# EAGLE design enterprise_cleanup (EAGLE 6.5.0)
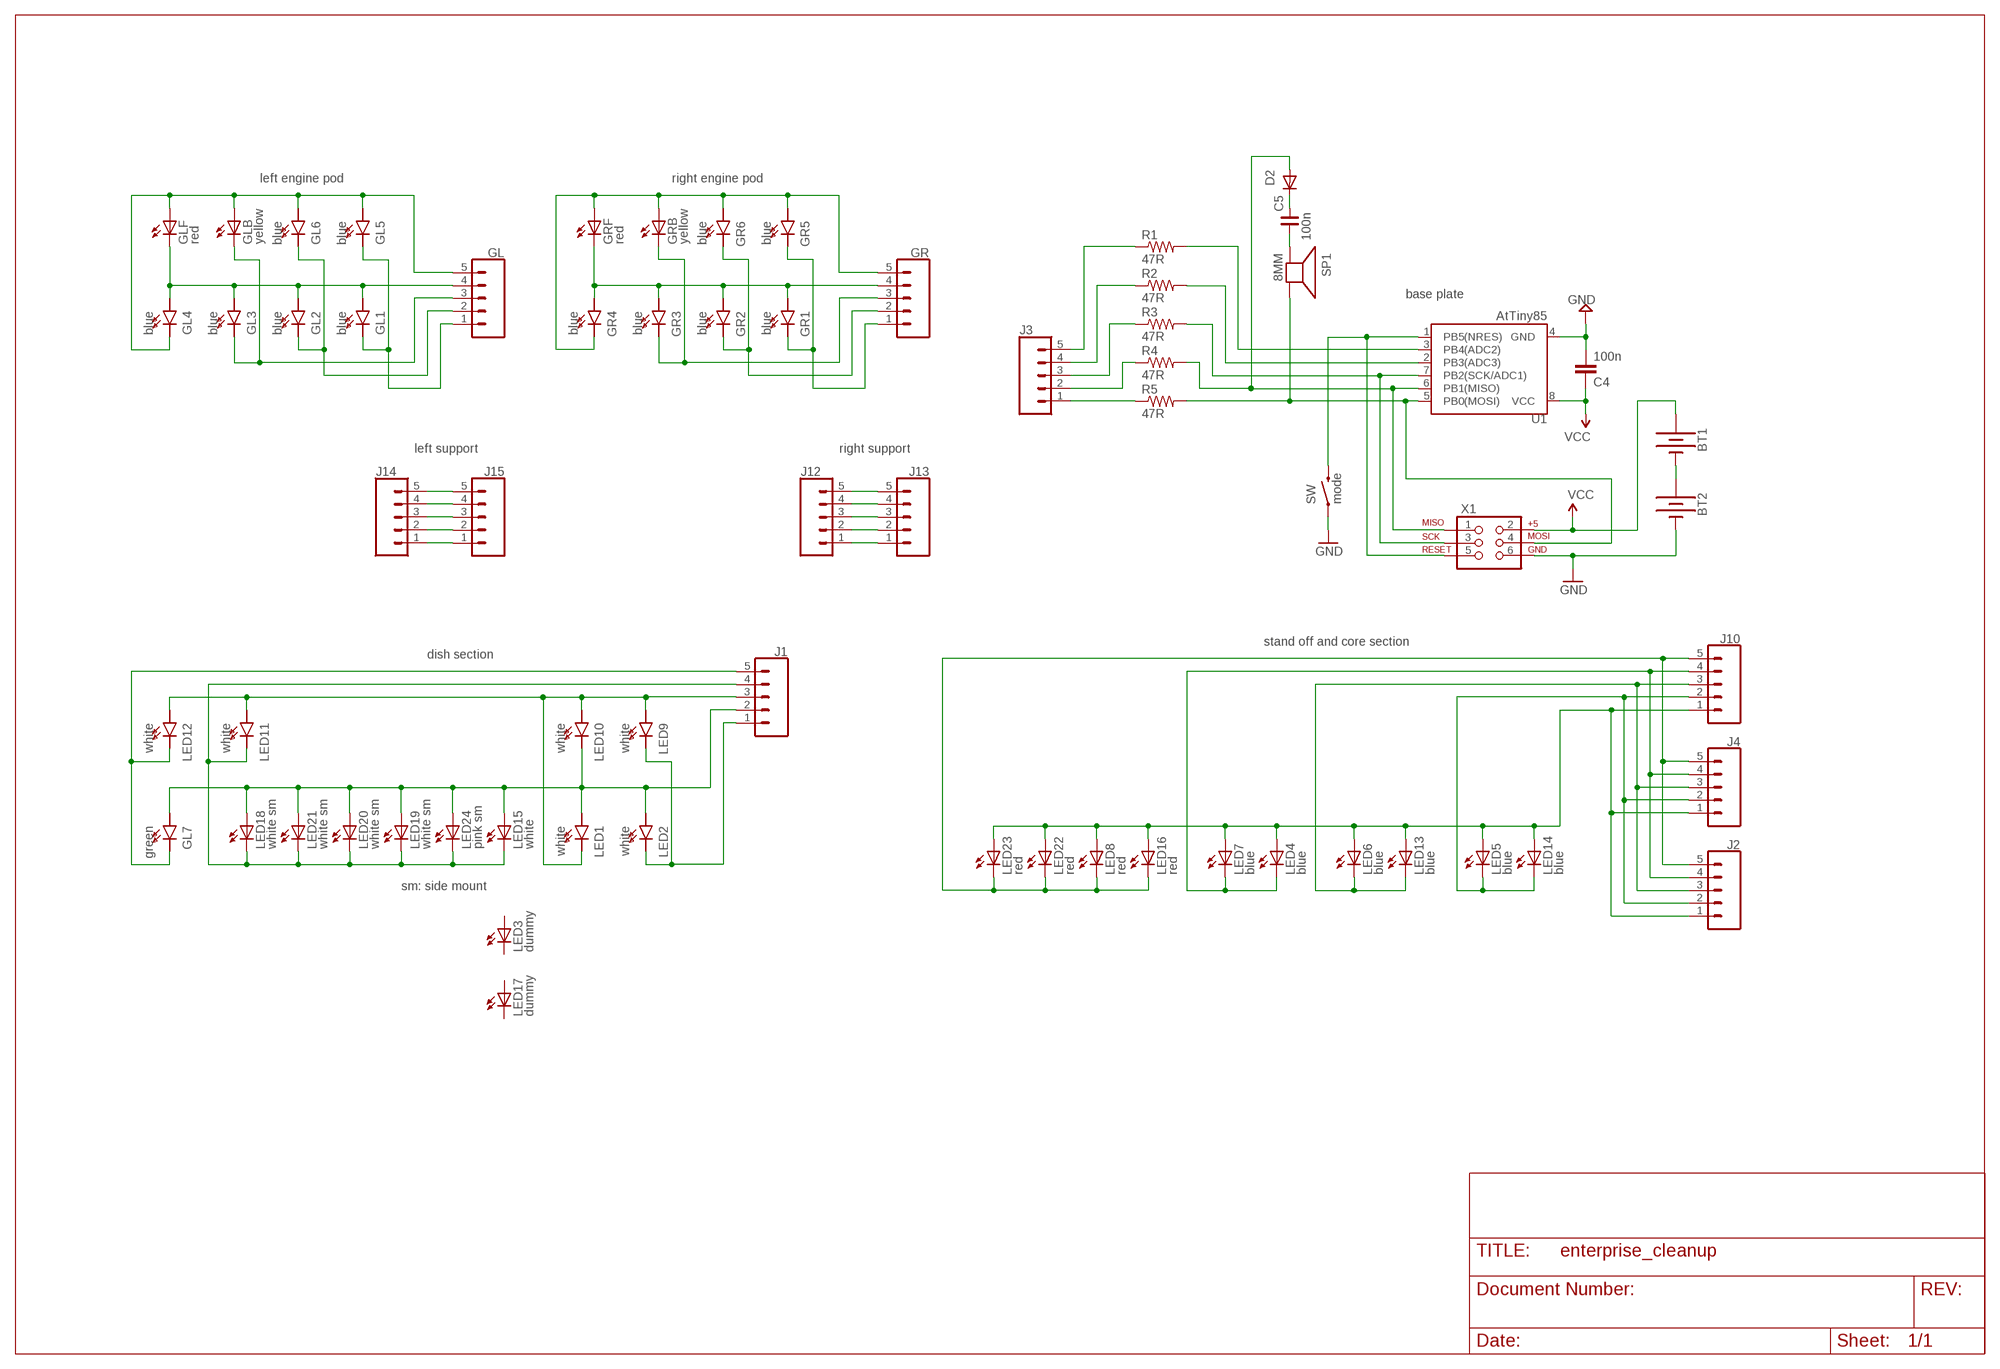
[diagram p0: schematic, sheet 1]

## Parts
BT1  BATTERY-AAA_KIT  [BATTERY-AAA-KIT]
BT2  BATTERY-AAA_KIT  [BATTERY-AAA-KIT]
C4  100n  CAP0603-CAP  [0603-CAP]
C5  100n  C_0603  [C0603]
D2  DIODESOD  [SOD-323]
GL  CONN_05NO_SILK  [1X05_NO_SILK]
GL1  blue  LED4014_SEGMENT3  [LED_4014_SEGMENT3]
GL2  blue  LED4014_SEGMENT3  [LED_4014_SEGMENT3]
GL3  blue  LED4014_SEGMENT3  [LED_4014_SEGMENT3]
GL4  blue  LED4014_SEGMENT3  [LED_4014_SEGMENT3]
GL5  blue  LED4014_SEGMENT3  [LED_4014_SEGMENT3]
GL6  blue  LED4014_SEGMENT3  [LED_4014_SEGMENT3]
GL7  green  LED4014_SEG_TRIANGLE  [LED_4014_SEGMENT2]
GLB  yellow  LEDCHIPLED_0805  [CHIPLED_0805]
GLF  red  LEDCHIPLED_0805  [CHIPLED_0805]
GR  CONN_05NO_SILK  [1X05_NO_SILK]
GR1  blue  LED4014_SEGMENT3  [LED_4014_SEGMENT3]
GR2  blue  LED4014_SEGMENT3  [LED_4014_SEGMENT3]
GR3  blue  LED4014_SEGMENT3  [LED_4014_SEGMENT3]
GR4  blue  LED4014_SEGMENT3  [LED_4014_SEGMENT3]
GR5  blue  LED4014_SEGMENT3  [LED_4014_SEGMENT3]
GR6  blue  LED4014_SEGMENT3  [LED_4014_SEGMENT3]
GRB  yellow  LEDCHIPLED_0805  [CHIPLED_0805]
GRF  red  LEDCHIPLED_0805  [CHIPLED_0805]
J1  CONN_05PTH_LONGPADS  [1X05_LONGPADS]
J2  CONN_05PTH_LONGPADS  [1X05_LONGPADS]
J3  CONN_05PTH_LONGPADS  [1X05_LONGPADS]
J4  CONN_05PTH_LONGPADS  [1X05_LONGPADS]
J10  CONN_05PTH_LONGPADS  [1X05_LONGPADS]
J12  CONN_05PTH_LONGPADS  [1X05_LONGPADS]
J13  CONN_05PTH_LONGPADS  [1X05_LONGPADS]
J14  CONN_05PTH_LONGPADS  [1X05_LONGPADS]
J15  CONN_05PTH_LONGPADS  [1X05_LONGPADS]
LED1  white  LED4014_SEGMENT3  [LED_4014_SEGMENT3]
LED2  white  LED4014_SEGMENT3  [LED_4014_SEGMENT3]
LED3  dummy  LED5MM  [LED5MM]
LED4  blue  LEDCHIPLED_0603  [CHIPLED_0603]
LED5  blue  LEDCHIPLED_0603  [CHIPLED_0603]
LED6  blue  LEDCHIPLED_0603  [CHIPLED_0603]
LED7  blue  LEDCHIPLED_0603  [CHIPLED_0603]
LED8  red  LEDCHIPLED_0805  [CHIPLED_0805]
LED9  white  LED4014_SEGMENT3  [LED_4014_SEGMENT3]
LED10  white  LED4014_SEGMENT3  [LED_4014_SEGMENT3]
LED11  white  LED4014_SEGMENT3  [LED_4014_SEGMENT3]
LED12  white  LED4014_SEGMENT3  [LED_4014_SEGMENT3]
LED13  blue  LEDCHIPLED_0603  [CHIPLED_0603]
LED14  blue  LEDCHIPLED_0603  [CHIPLED_0603]
LED15  white  LED5MM  [LED5MM]
LED16  red  LEDCHIPLED_0805  [CHIPLED_0805]
LED17  dummy  LED5MM  [LED5MM]
LED18  white sm  LEDCHIPLED_0805  [CHIPLED_0805]
LED19  white sm  LEDCHIPLED_0805  [CHIPLED_0805]
LED20  white sm  LEDCHIPLED_0805  [CHIPLED_0805]
LED21  white sm  LEDCHIPLED_0805  [CHIPLED_0805]
LED22  red  LEDCHIPLED_0805  [CHIPLED_0805]
LED23  red  LEDCHIPLED_0805  [CHIPLED_0805]
LED24  pink sm  LEDCHIPLED_0805  [CHIPLED_0805]
R1  47R  RESISTOR0603-RES  [0603-RES]
R2  47R  RESISTOR0603-RES  [0603-RES]
R3  47R  RESISTOR0603-RES  [0603-RES]
R4  47R  RESISTOR0603-RES  [0603-RES]
R5  47R  RESISTOR0603-RES  [0603-RES]
SP1  8MM  SPEAKER_BUZZER5MM  [BUZZER_SMT_5MM]
SW  mode  SWITCH-MOMENTARY-2SMD-3  [TACTILE_SWITCH_SMD-3]
U1  AtTiny85  ATTINY45TINY85-20-SMT  [SO08-EIAJ]
X1  AVR_SPI_PRG_6NS  [2X3-NS]

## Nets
E0: J2.1 J4.1 J10.1 LED4.A LED5.A LED6.A LED7.A LED8.A LED13.A LED14.A LED16.A LED22.A LED23.A
E1: J2.2 J4.2 J10.2 LED5.C LED14.C
E2: J2.3 J4.3 J10.3 LED6.C LED13.C
E3: J2.4 J4.4 J10.4 LED4.C LED7.C
E4: J2.5 J4.5 J10.5 LED8.C LED16.C LED22.C LED23.C
G0: GL1.K(C) GL5.K(C) GL.1
G1: GL2.K(C) GL6.K(C) GL.2
G2: GL3.K(C) GL.3 GLB.C
G3: GL1.A GL2.A GL3.A GL4.A GL.4 GLF.C
G4: GL4.K(C) GL5.A GL6.A GL.5 GLB.A GLF.A
GND: BT2.GND@1(-) C4.2 SW.1 U1.4(GND) X1.6
LX1: J3.1 R5.1
LX2: J3.2 R4.1
LX3: J3.3 R3.1
LX4: J3.4 R2.1
LX5: J3.5 R1.1
N$2: BT1.GND@1(-) BT2.PWR@1(+)
N$4: J12.1 J13.1
N$11: J12.2 J13.2
N$12: J12.3 J13.3
N$13: J12.4 J13.4
N$14: J12.5 J13.5
N$15: J14.1 J15.1
N$16: J14.2 J15.2
N$17: J14.3 J15.3
N$18: J14.4 J15.4
N$19: J14.5 J15.5
N$20: C5.2 D2.1(C)
N$21: C5.1 SP1.+
N$27: GR4.K(C) GR5.A GR6.A GR.5 GRB.A GRF.A
N$28: GR1.A GR2.A GR3.A GR4.A GR.4 GRF.C
N$29: GR3.K(C) GR.3 GRB.C
N$30: GR2.K(C) GR6.K(C) GR.2
N$31: GR1.K(C) GR5.K(C) GR.1
PB0: R5.2 SP1.- U1.5(PB0(MOSI)) X1.4
PB1: D2.2(A) R4.2 U1.6(PB1(MISO)) X1.1
PB2: R3.2 U1.7(PB2(SCK/ADC1)) X1.3
PB3: R2.2 U1.2(PB3(ADC3))
PB4: R1.2 U1.3(PB4(ADC2))
RESET: SW.4 U1.1(PB5(NRES)) X1.5
T0: J1.1 LED2.K(C) LED9.K(C)
T1: GL7.A J1.2 LED1.A LED2.A LED10.K(C) LED15.A LED18.A LED19.A LED20.A LED21.A LED24.A
T2: J1.3 LED1.K(C) LED9.A LED10.A LED11.A LED12.A
T3: J1.4 LED11.K(C) LED15.K(C) LED18.C LED19.C LED20.C LED21.C LED24.C
T4: GL7.K(C) J1.5 LED12.K(C)
VCC [pwr]: BT1.PWR@1(+) C4.1 U1.8(VCC) X1.2
Unconnected: LED3.A LED3.K(C) LED17.A LED17.K(C)

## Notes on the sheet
- left engine pod | right engine pod
- base plate
- left support | right support
- stand off and core section
- dish section
- sm: side mount

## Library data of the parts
BT1 BT2 = SparkFun-Batteries:BATTERY: Battery - Single Cell; PROD_ID: BATT-08571; SF_SKU: PRT-12718
C4 = SparkFun:CAP: Capacitor
C5 = rc-master-smd:C_: NON-POLARIZED CAP
D2 = SparkFun:DIODE: Diode
GL GR J1-J4 J10 J12-J15 = SparkFun-Connectors:CONN_05: Multi connection point. Often used as Generic Header-pin footprint for 0.1 inch spaced/style header connections On any of the 0.1 inch spaced packages, you can populate with these: Break Away Headers - Straight (PRT-00116) Break Away Male Headers - Right Angle (PRT-00553) Female Headers (PRT-00115)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
GL1-GL7 GR1-GR6 LED1 LED2 LED9-LED12 = yg_custom.5.5:LED
GLB GLF GRB GRF LED3-LED8 LED13-LED24 = led:LED: LED
R1-R5 = SparkFun:RESISTOR: Resistor
SP1 = microbuilder:SPEAKER: SPEAKER
SW = SparkFun-Electromechanical:SWITCH-MOMENTARY-2: Various NO switches- pushbuttons, reed, etc
U1 = SparkFun-DigitalIC:ATTINY45: Atmel 8-pin 2/4/8kB flash uC; PROD_ID: IC-09092; VALUE: Tiny85-20-SMT
X1 = SparkFun:AVR_SPI_PRG_6: AVR ISP 6 Pin This is the reduced ISP connector for AVR programming. Common on Arduino. This footprint will take up less PCB space and can be used with a 10-pin to 6-pin adapter such as SKU: BOB-08508

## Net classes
0 default: width 0.254 mm, drill 0.356 mm, clearance 0.381 mm
1 GNDa: width 0.254 mm, drill 0.356 mm, clearance 0.381 mm
2 pwr: width 0.254 mm, drill 0.356 mm, clearance 0.381 mm

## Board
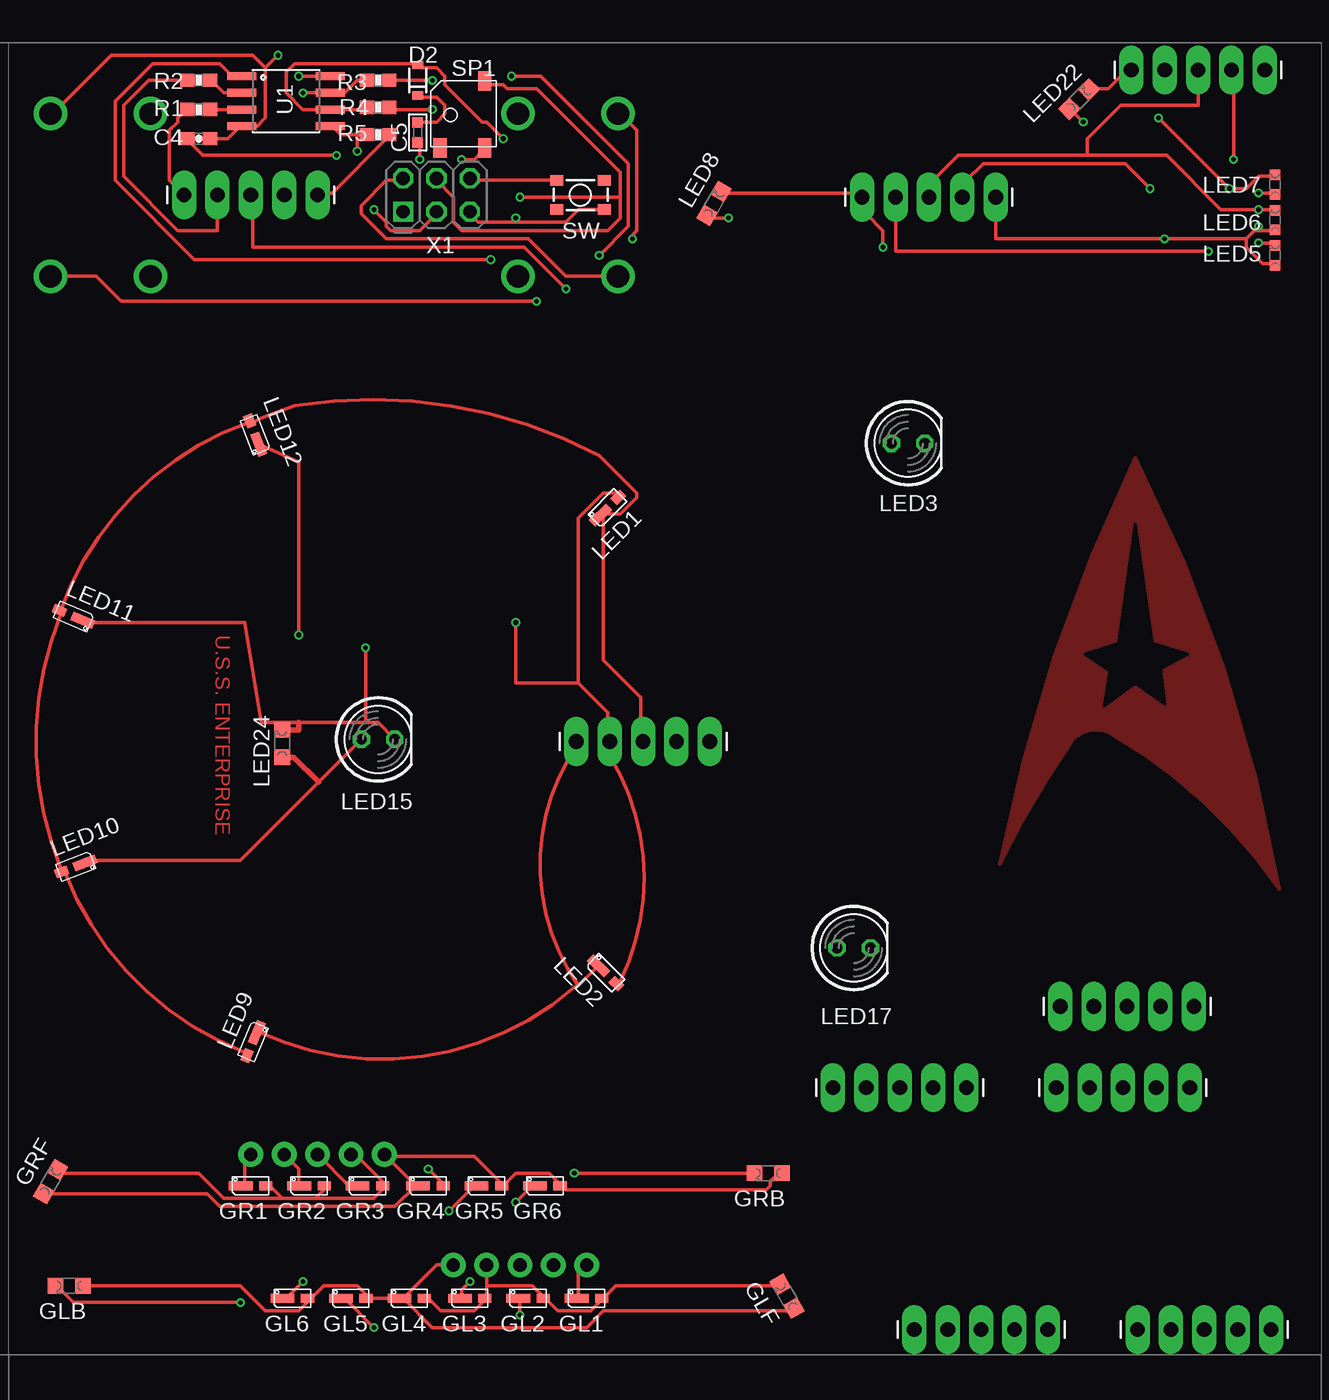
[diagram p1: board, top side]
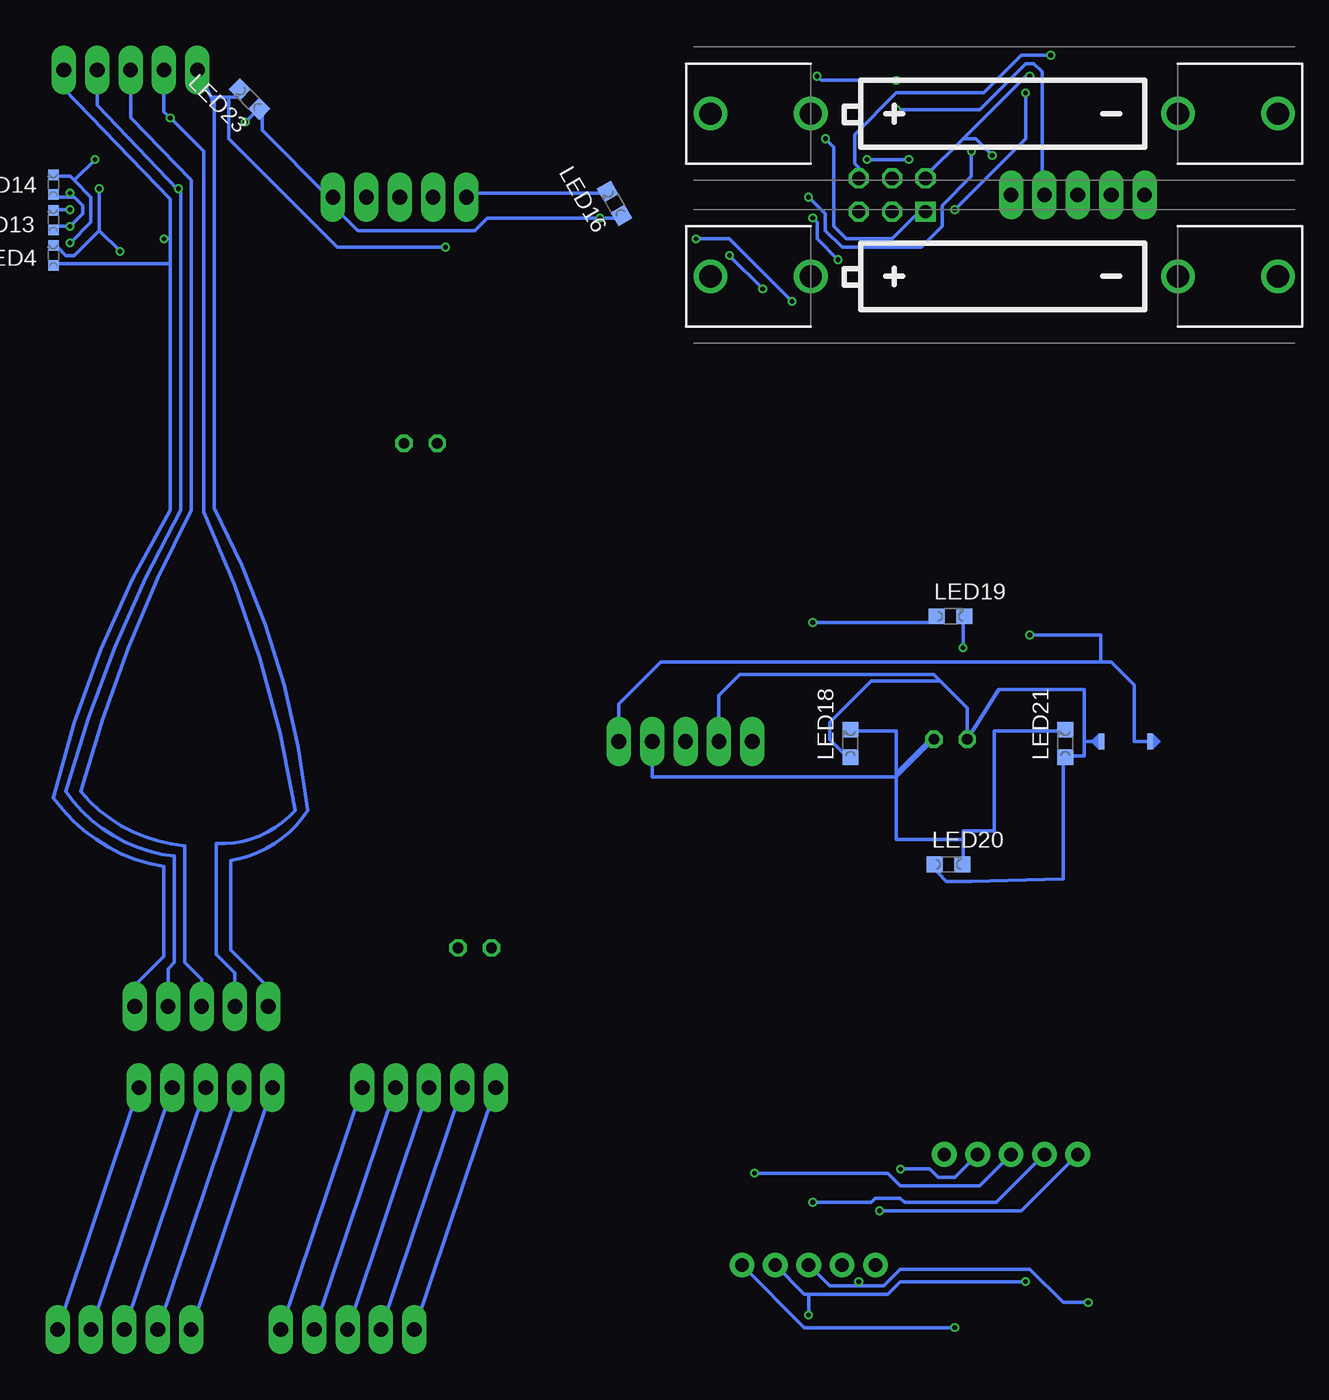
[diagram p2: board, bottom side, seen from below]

No outline drawn. Coordinates in mm, seen from the top.
Copper layers (1*16): Top 0.035mm / dielectric 1.5mm / Bottom 0.035mm
Design rules "ITEADstudio_DRC *": minimum track width 6mil, minimum drill 12mil, track to track 6mil, track to pad 6mil, pad to pad 6mil, via to via 6mil, smd to smd 0mil, copper to edge 20mil, drill to drill 8mil, minimum pad ring 10mil, minimum via ring 6mil, stop-mask expansion 2mil, vias tented up to drill 100mil, thermal gap 10mil
tRestrict: area 187.5,72.4 to 195.3,86.2

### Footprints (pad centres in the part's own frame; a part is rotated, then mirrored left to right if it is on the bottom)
BATTERY-AAA-KIT = drill 1.702: GND@1 21.59,0; GND@2 13.97,0; PWR@1 -21.59,0; PWR@2 -13.97,0
0603-CAP = smd 1.1 x 1: 1 -0.85,0; 2 0.85,0
C0603 = smd 0.8 x 0.8: 1 -0.762,0; 2 0.762,0
SOD-323 = smd 0.63 x 0.83: 1 -1.15,0; 2 1.15,0
1X05_NO_SILK = drill 1.016 pad 1.88: 1 0,0; 2 2.54,0; 3 5.08,0; 4 7.62,0; 5 10.16,0
LED_4014_SEGMENT3 = smd 1 x 0.7: A -1.143,0 | smd 1.8 x 0.7: K 0.762,0
LED_4014_SEGMENT2 = smd 0.4 x 1.2: A -1.85,0; K 1.85,0
CHIPLED_0805 = smd 1.2 x 1.2: A 0,-1.05; C 0,1.05
1X05_LONGPADS = drill 1.118 pad 1.88 long: 1 0,0; 2 2.54,0; 3 5.08,0; 4 7.62,0; 5 10.16,0
LED5MM = drill 0.813 octagon: A -1.27,0; K 1.27,0
CHIPLED_0603 = smd 0.8 x 0.8: A 0,-0.75; C 0,0.75
0603-RES = smd 1.1 x 1: 1 -0.85,0; 2 0.85,0
BUZZER_SMT_5MM = smd 1.5 x 1: + -2.6,-1.6; - 2.5,-1.6; MT -2.6,1.8
TACTILE_SWITCH_SMD-3 = smd 1 x 0.8: 1 -1.8,1.1; 2 1.8,1.1; 3 -1.8,-1.1; 4 1.8,-1.1
SO08-EIAJ = smd 0.61 x 2.21: 1 -1.905,-3.378; 2 -0.635,-3.378; 3 0.635,-3.378; 4 1.905,-3.378; 5 1.905,3.353; 6 0.635,3.353; 7 -0.635,3.353; 8 -1.905,3.353
2X3-NS = drill 1.016 square: 1 -2.54,-1.27 | drill 1.016 octagon: 2 -2.54,1.27; 3 0,-1.27; 4 0,1.27; 5 2.54,-1.27; 6 2.54,1.27

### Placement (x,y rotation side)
BT1  130.33,105.09 0 bottom
BT2  130.33,117.47 0 bottom
C4  120.02,115.57 0 top
C5  136.68,116.05 90 top
D2  136.68,120.02 90 top
GL  149.54,29.84 0 bottom
GL1  149.54,27.3 180 top
GL2  145.1,27.3 180 top
GL3  140.65,27.3 180 top
GL4  136.05,27.3 180 top
GL5  131.6,27.3 180 top
GL6  127.16,27.3 180 top
GL7  120.33,69.69 0 bottom
GLB  110.17,28.26 90 top
GLF  164.78,27.46 30 top
GR  123.98,38.26 0 top
GR1  123.98,35.88 180 top
GR2  128.43,35.88 180 top
GR3  132.87,35.88 180 top
GR4  137.48,35.88 180 top
GR5  141.92,35.88 180 top
GR6  146.37,35.88 180 top
GRB  163.35,36.83 90 top
GRF  108.74,36.2 330 top
J1  148.75,69.69 0 top
J2  195.74,49.53 180 top
J3  129.06,111.28 180 top
J4  180.66,111.12 180 top
J10  201.14,120.81 180 top
J12  201.61,24.92 180 top
J13  195.42,43.34 180 top
J14  184.63,24.92 180 top
J15  178.44,43.34 180 top
LED1  151.13,87.47 225 top
LED2  150.97,52.07 135 top
LED3  173.99,92.39 0 top
LED4  201.93,106.68 0 bottom
LED5  201.93,106.68 0 top
LED6  201.93,109.38 0 top
LED7  201.93,112.08 0 top
LED8  159.23,110.65 330 top
LED9  124.14,46.83 67 top
LED10  110.65,60.17 21 top
LED11  110.49,79.22 337 top
LED12  124.3,93.03 291 top
LED13  201.93,109.38 0 bottom
LED14  201.93,112.08 0 bottom
LED15  133.67,69.85 0 top
LED16  159.23,110.65 30 bottom
LED17  169.86,53.98 0 top
LED18  141.29,69.53 0 bottom
LED19  133.67,79.22 270 bottom
LED20  133.83,60.33 270 bottom
LED21  124.94,69.53 0 bottom
LED22  187.01,118.59 315 top
LED23  187.01,118.59 45 bottom
LED24  126.36,69.53 0 top
R1  120.02,117.79 0 top
R2  120.02,120.02 0 top
R3  133.67,120.02 180 top
R4  133.67,117.95 180 top
R5  133.67,115.89 180 top
SP1  140.18,117.47 90 top
SW  149.07,111.28 0 top
U1  126.68,118.43 270 top
U$1  [A4L-LOC]  34.13,-28.26 0 top
X1  138.11,111.28 0 top

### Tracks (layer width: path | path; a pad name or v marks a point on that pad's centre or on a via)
E0  (via drill 0.36)
  Top 0.254: v200.66,111.44 201.93,111.44 LED14.A | 199.71,107.95 199.71,107.31 200.98,106.05 201.93,106.05 LED4.A | 199.71,107.95 200.34,108.58 200.66,108.58 | 200.66,108.58 201.93,108.58 LED13.A | v160.34,109.54 158.43,109.54 LED16.A | 199.71,107.95 v193.52,107.95 180.66,107.95 J4.1 | 200.66,108.58 v200.66,108.9 | v187.32,116.84 186.69,117.47 LED23.A
  Bottom 0.254: J2.1 195.74,51.12 193.52,53.34 193.52,60.17 arc45 201.93,65.41 arc17 193.04,87.31 193.04,106.05 | 193.04,106.05 193.04,107.95 | 193.04,107.95 193.04,110.97 201.14,119.38 J10.1 | 193.04,106.05 201.93,106.05 LED4.A | 200.66,111.12 201.93,111.12 LED14.A | 200.66,111.12 200.34,111.12 199.71,110.49 199.71,109.86 v200.66,108.9 201.93,108.9 LED13.A | 200.66,111.12 v200.66,111.44 | v160.34,109.54 158.43,109.54 LED16.A 158.75,109.54 168.91,109.54 169.86,108.58 178.75,108.58 180.66,110.49 J4.1 180.97,111.12 186.06,116.2 186.06,117.47 LED23.A 186.69,117.47 v187.32,116.84 | v193.52,107.95 193.04,107.95
E1  (via drill 0.36)
  Top 0.254: v200.66,107.63 201.93,107.63 LED5.C | v198.75,113.98 198.75,120.65 J10.2 | v192.41,111.76 190.5,113.67 179.71,113.67 178.44,112.39 178.44,111.12 J4.2
  Bottom 0.254: J2.2 193.2,52.39 192.72,52.86 192.72,60.96 arc49 200.98,65.88 arc14 192.25,87.31 192.25,111.44 192.48,111.69 | 192.48,111.69 198.6,118.11 J10.2 | v200.66,107.63 199.07,109.22 199.07,111.12 200.34,112.39 | 200.34,112.39 200.66,112.71 201.93,112.71 LED14.C | v198.75,113.98 200.34,112.39 | v192.41,111.76 192.48,111.69
E2  (via drill 0.36)
  Top 0.254: LED13.C 201.93,110.17 v200.66,110.17 197.8,110.17 193.68,114.3 187.64,114.3 | 187.64,114.3 187.64,115.57 190.18,118.11 196.06,118.11 J10.3 | 187.64,114.3 177.8,114.3 175.9,112.39 175.9,111.12 J4.3
  Bottom 0.254: J2.3 190.66,51.59 191.93,52.86 191.93,61.75 arc45 199.87,65.88 arc12 191.45,87.31 191.45,112.39 196.06,117.16 J10.3 | v200.66,110.17 201.93,110.17 LED13.C
E3  (via drill 0.36)
  Top 0.254: LED7.C 201.93,112.71 200.66,112.71 199.71,111.76 v198.44,111.76 v193.04,117.16 | J4.4 173.04,107 v196.85,107
  Bottom 0.254: J2.4 188.12,52.07 189.55,53.5 189.55,61.91 arc-51 183.51,64.45 arc-16 190.5,87.15 190.5,114.62 v193.04,117.16 193.52,117.63 J10.4 | 198.44,108.58 200.34,106.68 200.98,106.68 201.61,107.31 201.93,107.31 LED4.C | v198.44,111.76 198.44,108.58 | 198.44,108.58 v196.85,107
E4  (via drill 0.36)
  Top 0.254: LED16.C 160.02,111.44 170.18,111.44 J4.5 170.81,111.12 170.81,109.86 172.09,108.58 v172.09,107.31 | LED23.C 187.96,119.38 189.23,119.38 190.5,120.65 J10.5
  Bottom 0.254: J2.5 185.58,50.96 188.44,53.82 188.44,60.64 arc-48 182.56,64.45 arc-22 189.71,87.47 189.71,118.27 189.8,118.46 | 189.8,118.46 189.93,118.71 | 189.93,118.71 J10.5 | LED16.C 160.02,111.44 170.18,111.44 J4.5 | 189.87,118.43 189.8,118.46 | 188.59,118.75 189.87,118.75 189.93,118.71 | 188.59,118.75 187.96,118.75 LED23.C | 188.59,118.75 188.59,115.57 180.34,107.31 v172.09,107.31
G0  (via drill 0.36)
  Top 0.254: v133.35,25.08 131.13,27.3 GL5.K | GL.1 148.91,29.21 148.91,27.3 GL1.K
  Bottom 0.254: v133.35,25.08 144.78,25.08 GL.1
G1  (via drill 0.36)
  Top 0.254: v127.95,28.57 126.68,27.3 GL6.K | v144.46,26.04 144.46,27.3 GL2.K
  Bottom 0.254: v127.95,28.57 137.48,28.57 138.43,27.62 144.46,27.62 | 144.46,27.62 144.78,27.62 GL.2 | 144.46,27.62 v144.46,26.04
G2  (via drill 0.36)
  Top 0.254: v123.19,26.99 110.49,26.99 109.22,28.26 GLB.C | v140.65,28.57 140.02,27.94 140.02,27.3 GL3.K
  Bottom 0.254: v123.19,26.99 125.09,26.99 127.64,29.53 137.48,29.53 138.75,28.26 140.65,28.26 | 140.65,28.26 142.88,28.26 GL.3 | 140.65,28.26 v140.65,28.57
G3
  Top 0.254: 141.92,27.3 140.97,26.35 138.43,26.35 137.48,27.3 GL4.A | GL.4 141.92,28.26 | 141.92,28.26 141.92,27.3 | 141.92,27.3 GL3.A | 146.37,27.3 147.32,26.35 149.86,26.35 150.81,27.3 | 150.81,27.3 151.76,28.26 164.15,28.26 GLF.C | 150.81,27.3 GL1.A | 141.92,28.26 145.41,28.26 146.37,27.3 | 146.37,27.3 GL2.A
G4
  Top 0.254: 128.59,27.3 129.54,28.26 132.08,28.26 133.03,27.3 | GLB.A 123.19,28.26 125.09,26.35 127.64,26.35 128.59,27.3 | 128.59,27.3 GL6.A | 135.57,27.3 137.79,25.08 149.54,25.08 150.81,26.35 165.1,26.35 GLF.A | GL.5 138.11,29.84 135.57,27.3 | 135.57,27.3 GL4.K 133.03,27.3 | 133.03,27.3 GL5.A
GND  (via drill 0.36)
  Top 0.254: SW.1 147,112.39 140.65,112.39 X1.6 | C4.2 122.24,115.57 123.19,116.52 U1.4 124.46,116.52 125.09,117.16 125.09,120.97 | 125.09,120.97 124.14,121.92 113.35,121.92 108.9,117.47 BT2.GND@1 | 125.09,120.97 v126.05,121.92
  Bottom 0.254: X1.6 140.65,113.35 140.97,113.67 140.97,115.89 137.79,119.06 131.13,119.06 128.27,121.92 v126.05,121.92
LX1
  Top 0.254: R5.1 134.3,115.89 134.3,115.57 130.18,111.44 129.22,111.44 J3.1
LX2  (via drill 0.36)
  Top 0.254: v137.79,117.79 134.62,117.79 R4.1
  Bottom 0.254: v137.79,117.79 131.44,117.79 127.95,121.28 127.32,121.28 126.68,120.65 126.68,111.44 J3.2
LX3  (via drill 0.36)
  Top 0.254: v137.79,120.02 R3.1 | v143.83,120.33 146.05,120.33 152.72,113.67 152.72,108.9 v150.5,106.68 | v147.96,104.14 144.78,107.31 124.14,107.31 124.14,111.12 J3.3
  Bottom 0.254: v137.79,120.02 143.51,120.02 v143.83,120.33 | v147.96,104.14 v150.5,106.68
LX4
  Top 0.254: R2.1 116.2,120.02 114.3,118.11 114.3,112.71 118.43,108.58 121.44,108.58 J3.4
LX5
  Top 0.254: J3.5 117.79,112.39 117.79,116.2 118.43,116.84 118.43,117.16 119.06,117.79 R1.1
N$2  (via drill 0.36)
  Top 0.254: BT1.GND@1 112.24,105.09 114.14,103.19 v145.73,103.19 | v153.03,107.95 153.03,108.27 153.35,108.58 153.35,116.2 152.08,117.47 BT2.PWR@1
  Bottom 0.254: v145.73,103.19 150.5,107.95 v153.03,107.95
N$4
  Bottom 0.254: J12.1 J13.1
N$9
  pour Top: 180.97,60.33 arc-15 191.29,91.28 arc-17 202.25,58.42 arc25 189.39,70.33 arc70 186.53,69.85 arc9
N$11
  Bottom 0.254: J12.2 J13.2
N$12
  Bottom 0.254: J12.3 J13.3
N$13
  Bottom 0.254: J12.4 J13.4
N$14
  Bottom 0.254: J12.5 J13.5
N$15
  Bottom 0.254: J14.1 J15.1
N$16
  Bottom 0.254: J14.2 J15.2
N$17
  Bottom 0.254: J14.3 J15.3
N$18
  Bottom 0.254: J14.4 J15.4
N$19
  Bottom 0.254: J14.5 J15.5
N$20
  Top 0.254: C5.2 136.84,116.84 138.11,116.84 138.75,117.47 138.75,118.11 138.11,118.75 136.84,118.75 D2.1
N$21  (via drill 0.36)
  Top 0.254: v136.84,113.98 136.84,115.25 C5.1 | v140.02,113.98 140.97,113.98 141.6,114.62 SP1.+
  Bottom 0.254: v140.02,113.98 v136.84,113.98
N$27
  Top 0.254: 147.64,35.88 146.69,36.83 144.15,36.83 143.19,35.88 GR5.A 142.88,35.88 142.88,36.2 140.97,38.1 134.3,38.1 | 147.64,35.88 147.96,35.56 163.19,35.56 163.51,35.88 163.51,36.2 164.15,36.83 GRB.A | 147.64,35.88 GR6.A | 136.53,35.88 134.94,34.29 121.6,34.29 120.65,35.24 108.27,35.24 GRF.A | 136.53,35.88 134.3,38.1 | 136.53,35.88 GR4.K | 134.3,38.1 GR.5
N$28  (via drill 0.36)
  Top 0.254: 133.99,35.88 133.99,36.2 131.76,38.42 GR.4 | v137.48,37.15 138.43,36.2 138.43,35.88 GR4.A | 126.36,34.92 125.41,35.88 GR1.A | 128.91,34.92 126.36,34.92 | 128.91,34.92 129.86,35.88 GR2.A | 126.36,34.92 121.92,34.92 120.02,36.83 109.54,36.83 GRF.C | 133.99,35.88 133.99,35.56 133.35,34.92 128.91,34.92 | 133.99,35.88 GR3.A
  Bottom 0.254: v137.48,37.15 135.25,37.15 134.62,36.51 133.35,36.51 GR.4
N$29  (via drill 0.36)
  Top 0.254: v148.59,36.83 GRB.C | GR3.K 131.44,35.88 GR.3
  Bottom 0.254: v148.59,36.83 138.43,36.83 137.48,35.88 131.44,35.88 GR.3
N$30  (via drill 0.36)
  Top 0.254: GR.2 127.64,37.15 127.64,35.88 GR2.K | v144.15,34.61 145.41,35.88 GR6.K
  Bottom 0.254: v144.15,34.61 139.7,34.61 139.38,34.92 137.48,34.92 137.16,34.61 130.18,34.61 GR.2
N$31  (via drill 0.36)
  Top 0.254: GR.1 123.51,37.78 123.51,35.88 GR1.K | v139.06,33.97 140.97,35.88 GR5.K
  Bottom 0.254: v139.06,33.97 128.27,33.97 GR.1
PB0  (via drill 0.36)
  Top 0.254: 132.08,115.89 130.81,115.89 130.18,116.52 U1.5 | 132.08,115.89 R5.2 | 152.08,111.12 152.08,109.54 151.13,108.58 140.02,108.58 139.38,109.22 139.38,111.12 138.11,112.39 X1.4 | 152.08,111.12 152.08,113.03 145.73,119.38 143.51,119.38 143.19,119.7 141.92,119.7 SP1.- | v132.08,114.62 132.08,115.89 | 152.08,111.12 v144.46,111.12
  Bottom 0.254: v132.08,114.62 132.08,112.71 134.3,110.49 134.3,108.9 135.89,107.31 141.92,107.31 143.19,108.58 143.19,109.86 v144.46,111.12
PB1  (via drill 0.36)
  Top 0.254: R4.2 132.72,117.79 U1.6 127.95,117.79 126.68,119.06 126.68,120.65 127.32,121.28 136.53,121.28 D2.2 136.84,120.97 138.11,120.97 138.75,120.33 138.75,119.7 141.6,116.84 141.92,116.84 v143.19,115.57
  Bottom 0.254: v143.19,115.57 142.56,114.94 142.56,108.9 141.6,107.95 138.11,107.95 136.21,109.86 135.57,109.86 X1.1
PB2  (via drill 0.36)
  Top 0.254: R3.2 132.08,120.02 131.13,119.06 U1.7 v127.95,119.06 | v133.35,110.17 134.3,109.22 134.3,108.9 134.62,108.58 136.84,108.58 138.11,109.86 X1.3
  Bottom 0.254: v127.95,119.06 127.95,115.57 v133.35,110.17
PB3
  Top 0.254: U1.2 121.92,119.06 120.97,120.02 R2.2
PB4
  Top 0.254: U1.3 R1.2
RESET  (via drill 0.36)
  Top 0.254: 144.15,109.22 141.29,109.22 140.65,109.86 X1.5 | 144.15,109.22 147.96,109.22 148.91,110.17 150.81,110.17 SW.4 | U1.1 122.56,120.33 121.6,121.28 116.52,121.28 113.67,118.43 113.67,112.39 119.7,106.36 v142.24,106.36 | 144.15,109.22 v144.15,109.54
  Bottom 0.254: v142.24,106.36 143.83,107.95 143.83,109.22 v144.15,109.54
T0
  Top 0.254: 148.91,51.12 150.18,52.39 LED2.K | 148.91,51.12 148.59,50.96 arc-66 124.46,47.62 LED9.K | 148.91,51.12 arc-70 148.91,69.53 J1.1
T1  (via drill 0.36)
  Top 0.254: LED2.A 152.08,51.44 arc58 151.29,68.58 J1.2 151.13,69.85 151.13,71.91 148.91,74.14 | 148.91,74.14 148.91,86.68 150.81,88.58 151.76,88.58 LED1.A | LED15.A 129.14,66.6 123.19,60.64 111.44,60.64 LED10.K | 148.91,74.14 144.15,74.14 v144.15,78.74
  Top 0.406: LED24.A 127.26,68.48 129.14,66.6
  Bottom 0.254: GL7.A 123.51,69.69 | 134.54,74.37 132.4,72.23 LED15.A 130.02,73.66 123.51,73.66 123.51,69.69 | 134.54,74.37 134.94,74.77 149.7,74.77 151.29,73.18 J1.2 | 123.51,69.69 123.51,68.58 124.46,68.58 LED21.A 125.09,67.94 125.09,59.21 132.08,59.05 133.99,59.05 134.62,59.69 134.62,60.33 LED20.A | v144.15,78.74 135.25,78.74 LED19.A | LED18.A 141.6,68.58 142.88,69.85 142.88,71.12 139.7,74.3 134.62,74.3 134.54,74.37
T2
  Top 0.254: J1.3 153.67,69.85 153.67,73.03 150.81,75.88 150.81,86.68 LED1.K 150.81,87 152.08,87 153.35,88.27 153.35,88.58 150.5,91.44 arc37 127.32,95.25 124.78,94.3 124.14,93.98 LED12.A 123.83,93.98 arc51 109.54,79.69 LED11.A 109.54,79.38 arc45 109.54,60.01 LED10.A 109.86,59.69 arc47 123.51,46.04 LED9.A
T3  (via drill 0.36)
  Top 0.254: 132.72,71.12 133.67,71.12 LED15.K | 132.72,71.12 127.64,71.12 124.78,71.12 123.51,78.74 111.44,78.74 LED11.K | 132.72,71.12 v132.72,76.83
  Top 0.406: LED24.C 127.64,70.58 127.64,71.12
  Bottom 0.254: J1.4 156.37,66.99 137.79,66.99 LED15.K 135.25,69.85 137.79,67.31 | v132.72,76.83 132.72,78.74 LED19.C | 132.72,62.23 132.72,60.33 LED20.C | 132.72,62.23 132.72,62.87 130.33,62.87 130.33,70.48 125.09,70.48 LED21.C | 132.72,62.23 137.79,62.23 137.79,67.31 | 137.79,67.31 137.79,70.48 140.97,70.48 LED18.C
T4  (via drill 0.36)
  Top 0.254: v127.64,77.79 127.64,90.96 LED12.K
  Bottom 0.254: GL7.K 119.7,69.69 119.7,73.98 121.44,75.72 122.24,75.72 | 122.24,75.72 155.73,75.72 158.91,72.55 J1.5 | v127.64,77.79 122.24,77.79 122.24,75.72
VCC  (via drill 0.36)
  Top 0.254: v130.49,114.3 120.33,114.3 119.38,115.25 119.38,115.57 C4.1 | v127.64,120.33 U1.8 | BT1.PWR@1 147.96,105.09 145.1,107.95 134.3,107.95 132.4,109.86 132.4,110.49 134.3,112.39 135.57,112.39 X1.2
  Bottom 0.254: v130.49,114.3 131.76,115.57 132.72,115.57 | 132.72,115.57 135.57,112.71 X1.2 | v127.64,120.33 127.95,120.33 132.72,115.57

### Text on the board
Top: U.S.S. ENTERPRISE
tStop: U.S.S. ENTERPRISE
t_draw: boldly go ... | ENGAGE | U.S.S. ENTERPRISE | LED-/+ | LED+/- | NCC-1701 | NCC-1701
b_draw: U.S.S. ENTERPRISE | (Bobricius) - PeMi Technology / Factory For Materializing Dreams | + | www.youtube.com/bobricius / hackaday.io/bobricius / www.tindie.com/stores/bobricius/ / www.tindie.com/stores/kitsforkids/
